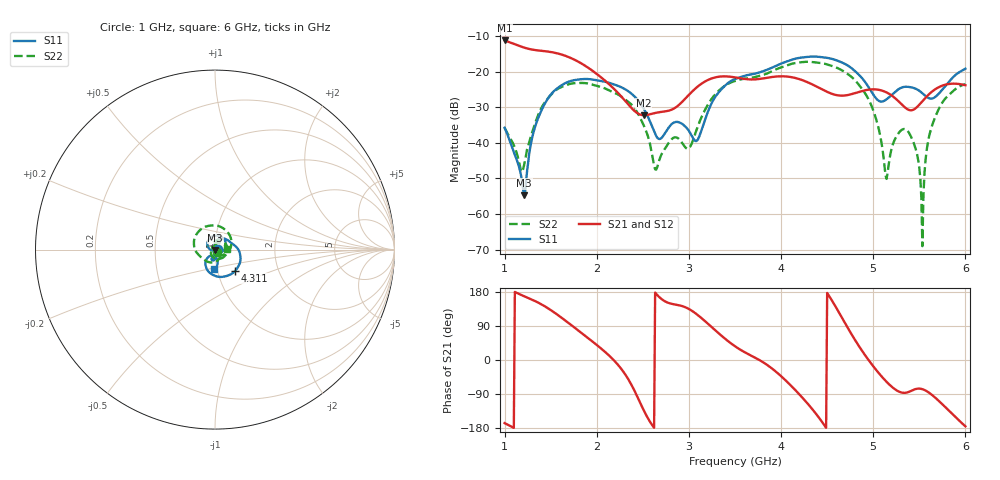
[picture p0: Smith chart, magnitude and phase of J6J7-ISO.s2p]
!Agilent Technologies,E8364B,MY43040528,A.07.50.67
!Agilent E8364B: A.07.50.67
!Date: Sunday, March 01, 2026 23:03:50
!Correction: S11(Full 2 Port(1,2))
!S21(Full 2 Port(1,2))
!S12(Full 2 Port(1,2))
!S22(Full 2 Port(1,2))
!S2P File: Measurements: S11, S21, S12, S22:
# Hz S  dB  R 50
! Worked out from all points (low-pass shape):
!   451 points, 1 GHz to 6 GHz, reference 50 ohm
!   highest |S21| = -11.18 dB at 1 GHz (marker M1); lowest = -32.2 dB at 2.511 GHz (marker M2)
!   |S21| within 3 dB of the highest: start of sweep to 1.432 GHz
!   lowest |S11| = -54.8 dB at 1.211 GHz (marker M3), VSWR 1.00, Z = 50.1 - j0.163 ohm
!   |S11| at or under -10 dB: start of sweep to end of sweep
!   |S22| runs from -69.0 to -17.2 dB; largest |S21 - S12| = 0.00096
!   S11 on the Smith chart (normalised r, x): 1 GHz: 1.03, +0.01; 4.311 GHz: 1.22, -0.29; 6 GHz: 0.96, -0.21
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1e9  -35.74 11.4  -11.18 -166.5  -11.21 -166.5  -35.79 -42.2
1.211111e9  -54.76 -63.0  -13.18 168.3  -13.21 168.3  -46.26 -146.1
1.311111e9  -37.22 -157.7  -13.80 157.7  -13.84 157.7  -36.04 154.0
1.433333e9  -29.11 168.2  -14.18 142.2  -14.21 142.2  -28.70 110.3
1.844444e9  -22.05 77.9  -17.82 69.4  -17.85 69.5  -23.13 -5.0
2.511111e9  -30.42 -24.5  -32.20 -133.4  -32.24 -133.4  -35.16 -171.3
2.666667e9  -38.78 2.3  -31.41 168.8  -31.44 168.8  -45.87 43.2
2.866667e9  -34.08 31.1  -29.83 145.8  -29.86 145.8  -38.48 -53.5
2.988889e9  -36.22 22.5  -26.76 136.0  -26.79 136.0  -41.65 -42.6
3.088889e9  -39.33 67.0  -24.28 119.9  -24.31 119.9  -35.88 -16.7
3.5e9  -22.03 52.2  -21.56 36.2  -21.59 36.3  -22.58 -104.6
4.311111e9  -15.75 -46.0  -23.21 -121.6  -23.24 -121.6  -17.20 110.8
4.344444e9  -15.70 -51.1  -23.62 -131.4  -23.65 -131.4  -17.27 103.4
4.877778e9  -21.75 -129.5  -25.40 24.6  -25.44 24.6  -24.79 -28.0
5.166667e9  -27.25 -92.9  -26.10 -62.9  -26.13 -63.0  -46.30 112.3
5.244444e9  -25.49 -92.0  -27.57 -78.7  -27.61 -78.7  -38.53 61.9
5.366667e9  -24.20 -101.2  -30.45 -85.7  -30.49 -85.7  -36.46 18.6
5.466667e9  -24.82 -110.2  -30.11 -76.2  -30.14 -76.2  -42.22 -20.1
5.533333e9  -26.02 -110.3  -28.26 -77.0  -28.29 -77.0  -69.03 35.4
5.588889e9  -27.21 -105.5  -26.70 -83.6  -26.74 -83.6  -40.51 121.3
5.655556e9  -27.35 -92.7  -25.21 -95.8  -25.24 -95.8  -33.84 103.2
6e9  -19.13 -94.0  -23.77 -175.0  -23.80 -175.1  -23.46 3.2
